(* Logix 5000 AddOnInstructionDefinition export YAI_Assy_166_22_23_EIP_Hz; software revision 17.00 *)

ADD_ON_INSTRUCTION YAI_Assy_166_22_23_EIP_Hz   (* revision 1.0, vendor Yaskawa America, Inc. *)
// YAI Assembly 166 and 22/23
// Help:
// This add-on instruction is for use with input assemblie 166 and output assemblies 116.
// Node_Input_Assy is defined as the node's input assembly integer array.
// Node_Output_Assy is defined as the node's output assembly integer array.
// Torque limit/reference, torque compensation and torque output variables are only available with A1000.
VAR_IN_OUT
   Node_Input_Assy : AB:ETHERNET_MODULE_INT_44Bytes:I:0; {required}   // Input assembly words
   Node_Output_Assy : AB:ETHERNET_MODULE_INT_6Bytes:O:0; {required}   // Output assembly words
END_VAR
VAR_INPUT
   RunFwd : BOOL; {visible}   // Forward run command
   RunRev : BOOL; {visible}   // Reverse run command
   FaultReset : BOOL; {visible}   // Fault reset command
   Freq_Ref : REAL; {visible}   // Frequency reference command in Hz (xx.xx resolution)
   Net_Ref : BOOL;   // Network reference control bit
   Net_Control : BOOL;   // Network start/stop control bit
END_VAR
VAR_OUTPUT
   Running : BOOL; {visible}   // Drive running forward status bit
   ZSP : BOOL; {visible}   // Drive zero speed status bit
   RunningRev : BOOL; {visible}   // Drive running reverse status bit
   Reset : BOOL; {visible}   // Drive reset command status bit
   At_Speed : BOOL; {visible}   // Drive at commanded speed status bit
   Ready : BOOL; {visible}   // Drive ready status bit
   Alarm : BOOL; {visible}   // Drive alarm status bit
   Faulted : BOOL; {visible}   // Drive faulted status bit
   OPE : BOOL;   // OPE alarm/fault present
   UV : BOOL;   // Drive in UV (undervoltage) state status bit
   NetCtrlStatus : BOOL; {visible}   // Drive network run source status bit (1 = source coming from network)
   MFO_1_Status : BOOL; {visible}   // Drive multi-function output 1 (M1-M2 for A/P1000, MA/MB/MC for V1000) status
   MFO_2_Status : BOOL; {visible}   // Drive multi-function output 1 (M3-M4 for A/P1000, P1 for V1000) status
   MFO_3_Status : BOOL; {visible}   // Drive multi-function output 1 (M5-M6 for A/P1000, P2 for V1000) status
   ZSV : BOOL; {visible}   // Drive zero servo completed status bit
   Motor_Speed : REAL; {visible}   // Motor speed in Hz (xx.xx resolution)
   Torque_Actual : REAL; {visible}   // Drive torque output in % (xxx.x resolution)
   PG_Count : INT;   // Encoder feedback count
   Freq_Cmd : REAL; {visible}   // Commanded frequency in Hz (xx.xx resolution)
   Output_Freq : REAL; {visible}   // Drive output frequency in Hz (xx.xx resolution)
   Output_Current : REAL; {visible}   // Drive output current in A (xxx.x resolution)
   Analog_Input_1_Level : REAL;   // Analog input 1 level in % (xxx.x resolution)
   DC_Bus_Volt : INT; {visible}   // DC bus voltage in Vdc (xxx resolution)
   Error_Code : INT;   // Custom input/output error code. Refer to custom error bit to determine which parameter error is pertaining to.
   Custom_In_1 : INT; {visible}   // Custom input 1 - F7-33
   Custom_In_2 : INT; {visible}   // Custom input 2 - F7-34
   Custom_In_3 : INT; {visible}   // Custom input 3 - F7-35
   Custom_In_4 : INT;   // Custom input 4 - F7-36
   Custom_In_5 : INT;   // Custom input 5 - F7-37
   Custom_In_6 : INT;   // Custom input 6 - F7-38
   Custom_In_7 : INT;   // Custom input 7 - F7-39
   Custom_In_8 : INT;   // Custom input 8 -F7-40
   Custom_In_9 : INT;   // Custom input 9 - F7-41
   Custom_In_10 : INT;   // Custom input 10 - F7-42
   Custom_In_1_Error : BOOL;   // Custom input 1 error bit
   Custom_In_2_Error : BOOL;   // Custom input 2 error bit
   Custom_In_3_Error : BOOL;   // Custom input 3 error bit
   Custom_In_4_Error : BOOL;   // Custom input 4 error bit
   Custom_In_5_Error : BOOL;   // Custom input 5 error bit
   Custom_In_6_Error : BOOL;   // Custom input 6 error bit
   Custom_In_7_Error : BOOL;   // Custom input 7 error bit
   Custom_In_8_Error : BOOL;   // Custom input 8 error bit
   Custom_In_9_Error : BOOL;   // Custom input 9 error bit
   Custom_In_10_Error : BOOL;   // Custom input 10 error bit
END_VAR
VAR_INPUT
   Motor_Rated_Torq : REAL;
   Torq_Ref_Limit : REAL;
END_VAR
VAR
   FRef_Convert : DINT;
   FOut_Convert : REAL;
   FOut_Temp : REAL;
   TRef_Convert : INT;
   TComp_Convert : INT;
   TOut_Convert : REAL;
   TOut_Temp : REAL;
   IOut_Temp : REAL;
   IOut_Convert : REAL;
   AO1_Convert : INT;
   AO2_Convert : INT;
   Motor_Speed_Temp : REAL;
   Motor_Speed_Convert : REAL;
   Freq_Cmd_Temp : REAL;
   Freq_Cmd_Convert : REAL;
   AI1_Temp : REAL;
   AI1_Convert : REAL;
   Motor_Torq_Temp : REAL;
END_VAR

ROUTINE Logic   (* ladder *)
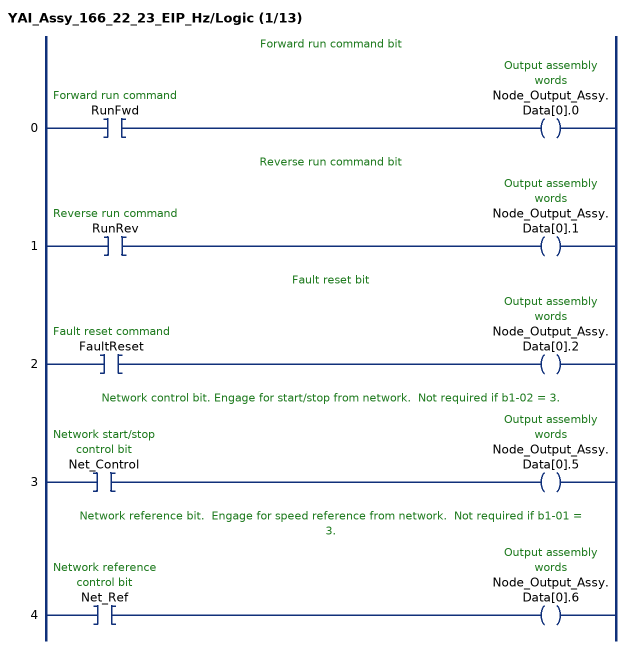
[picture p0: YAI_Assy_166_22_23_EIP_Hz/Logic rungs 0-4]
   // Forward run command bit
   0: XIC(RunFwd)OTE(Node_Output_Assy.Data[0].0);
   // Reverse run command bit
   1: XIC(RunRev)OTE(Node_Output_Assy.Data[0].1);
   // Fault reset bit
   2: XIC(FaultReset)OTE(Node_Output_Assy.Data[0].2);
   // Network control bit. Engage for start/stop from network.  Not required if b1-02 = 3.
   3: XIC(Net_Control)OTE(Node_Output_Assy.Data[0].5);
   // Network reference bit.  Engage for speed reference from network.  Not required if b1-01 = 3.
   4: XIC(Net_Ref)OTE(Node_Output_Assy.Data[0].6);
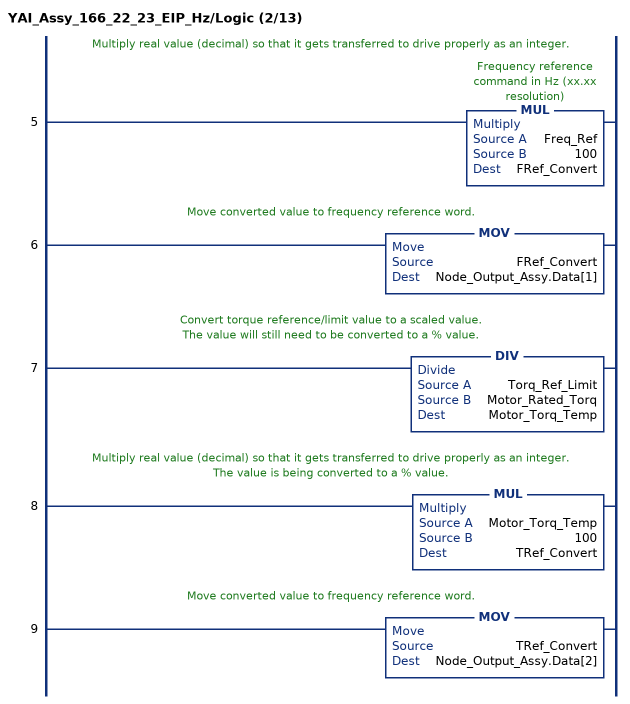
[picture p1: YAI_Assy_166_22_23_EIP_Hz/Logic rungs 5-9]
   // Multiply real value (decimal) so that it gets transferred to drive properly as an integer.
   5: MUL(Freq_Ref,100,FRef_Convert);
   // Move converted value to frequency reference word.
   6: MOV(FRef_Convert,Node_Output_Assy.Data[1]);
   // Convert torque reference/limit value to a scaled value.
   // The value will still need to be converted to a % value.
   7: DIV(Torq_Ref_Limit,Motor_Rated_Torq,Motor_Torq_Temp);
   // Multiply real value (decimal) so that it gets transferred to drive properly as an integer.
   // The value is being converted to a % value.
   8: MUL(Motor_Torq_Temp,100,TRef_Convert);
   // Move converted value to frequency reference word.
   9: MOV(TRef_Convert,Node_Output_Assy.Data[2]);
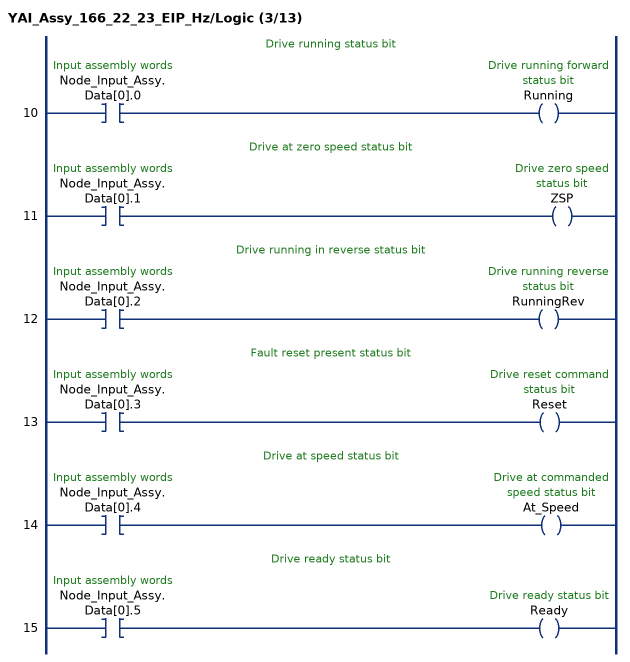
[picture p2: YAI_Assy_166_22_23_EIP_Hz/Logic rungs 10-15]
   // Drive running status bit
   10: XIC(Node_Input_Assy.Data[0].0)OTE(Running);
   // Drive at zero speed status bit
   11: XIC(Node_Input_Assy.Data[0].1)OTE(ZSP);
   // Drive running in reverse status bit
   12: XIC(Node_Input_Assy.Data[0].2)OTE(RunningRev);
   // Fault reset present status bit
   13: XIC(Node_Input_Assy.Data[0].3)OTE(Reset);
   // Drive at speed status bit
   14: XIC(Node_Input_Assy.Data[0].4)OTE(At_Speed);
   // Drive ready status bit
   15: XIC(Node_Input_Assy.Data[0].5)OTE(Ready);
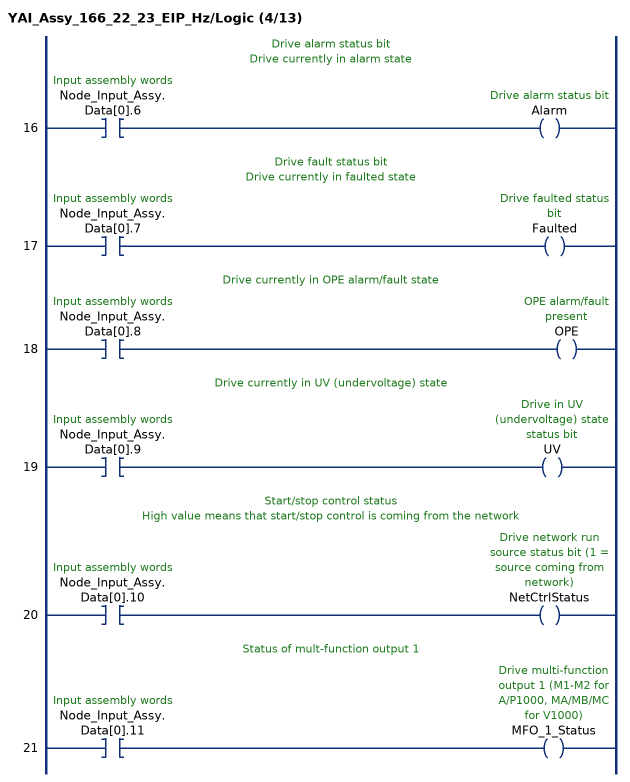
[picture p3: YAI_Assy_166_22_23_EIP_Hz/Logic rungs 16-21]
   // Drive alarm status bit
   // Drive currently in alarm state
   16: XIC(Node_Input_Assy.Data[0].6)OTE(Alarm);
   // Drive fault status bit
   // Drive currently in faulted state
   17: XIC(Node_Input_Assy.Data[0].7)OTE(Faulted);
   // Drive currently in OPE alarm/fault state
   18: XIC(Node_Input_Assy.Data[0].8)OTE(OPE);
   // Drive currently in UV (undervoltage) state
   19: XIC(Node_Input_Assy.Data[0].9)OTE(UV);
   // Start/stop control status
   // High value means that start/stop control is coming from the network
   20: XIC(Node_Input_Assy.Data[0].10)OTE(NetCtrlStatus);
   // Status of mult-function output 1
   21: XIC(Node_Input_Assy.Data[0].11)OTE(MFO_1_Status);
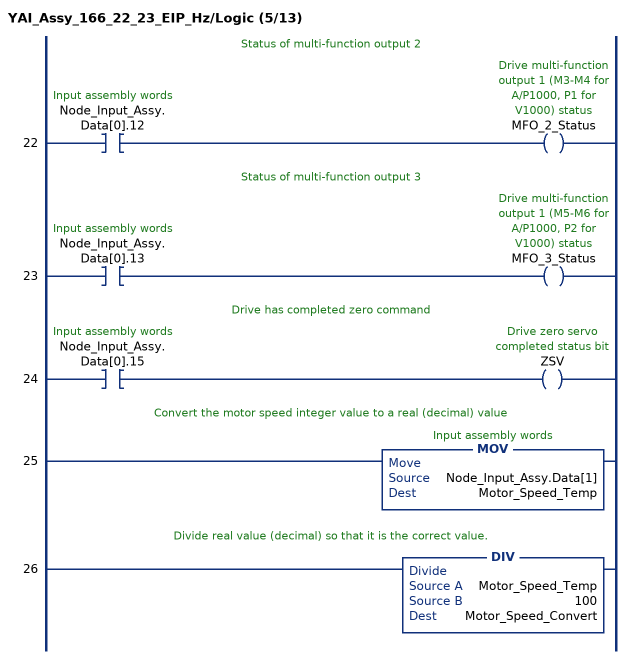
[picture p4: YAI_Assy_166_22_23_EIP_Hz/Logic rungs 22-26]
   // Status of multi-function output 2
   22: XIC(Node_Input_Assy.Data[0].12)OTE(MFO_2_Status);
   // Status of multi-function output 3
   23: XIC(Node_Input_Assy.Data[0].13)OTE(MFO_3_Status);
   // Drive has completed zero command
   24: XIC(Node_Input_Assy.Data[0].15)OTE(ZSV);
   // Convert the motor speed integer value to a real (decimal) value
   25: MOV(Node_Input_Assy.Data[1],Motor_Speed_Temp);
   // Divide real value (decimal) so that it is the correct value.
   26: DIV(Motor_Speed_Temp,100,Motor_Speed_Convert);
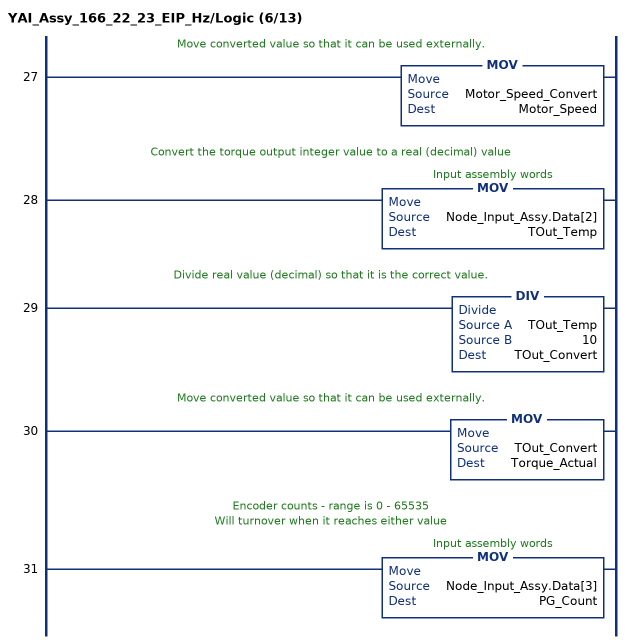
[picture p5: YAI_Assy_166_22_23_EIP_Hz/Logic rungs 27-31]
   // Move converted value so that it can be used externally.
   27: MOV(Motor_Speed_Convert,Motor_Speed);
   // Convert the torque output integer value to a real (decimal) value
   28: MOV(Node_Input_Assy.Data[2],TOut_Temp);
   // Divide real value (decimal) so that it is the correct value.
   29: DIV(TOut_Temp,10,TOut_Convert);
   // Move converted value so that it can be used externally.
   30: MOV(TOut_Convert,Torque_Actual);
   // Encoder counts - range is 0 - 65535
   // Will turnover when it reaches either value
   31: MOV(Node_Input_Assy.Data[3],PG_Count);
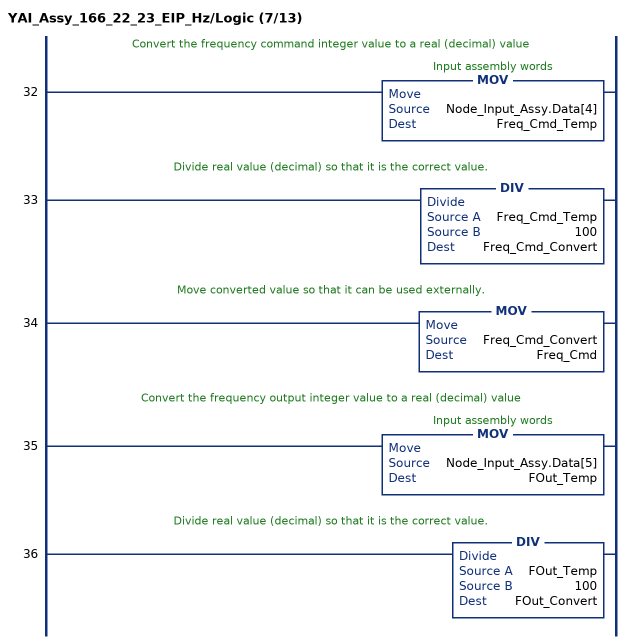
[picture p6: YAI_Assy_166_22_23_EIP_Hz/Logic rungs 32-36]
   // Convert the frequency command integer value to a real (decimal) value
   32: MOV(Node_Input_Assy.Data[4],Freq_Cmd_Temp);
   // Divide real value (decimal) so that it is the correct value.
   33: DIV(Freq_Cmd_Temp,100,Freq_Cmd_Convert);
   // Move converted value so that it can be used externally.
   34: MOV(Freq_Cmd_Convert,Freq_Cmd);
   // Convert the frequency output integer value to a real (decimal) value
   35: MOV(Node_Input_Assy.Data[5],FOut_Temp);
   // Divide real value (decimal) so that it is the correct value.
   36: DIV(FOut_Temp,100,FOut_Convert);
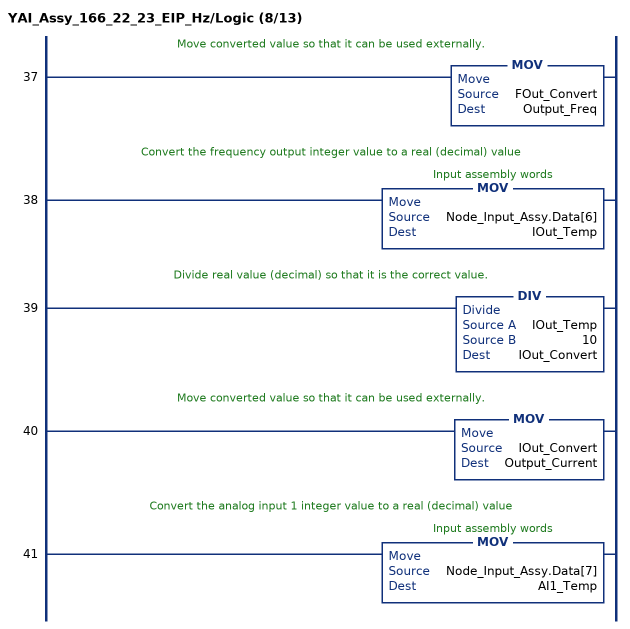
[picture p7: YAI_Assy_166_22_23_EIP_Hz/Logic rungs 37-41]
   // Move converted value so that it can be used externally.
   37: MOV(FOut_Convert,Output_Freq);
   // Convert the frequency output integer value to a real (decimal) value
   38: MOV(Node_Input_Assy.Data[6],IOut_Temp);
   // Divide real value (decimal) so that it is the correct value.
   39: DIV(IOut_Temp,10,IOut_Convert);
   // Move converted value so that it can be used externally.
   40: MOV(IOut_Convert,Output_Current);
   // Convert the analog input 1 integer value to a real (decimal) value
   41: MOV(Node_Input_Assy.Data[7],AI1_Temp);
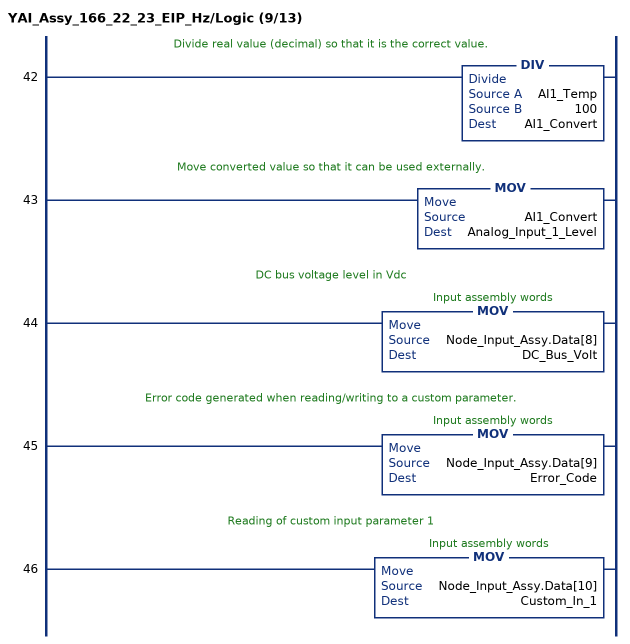
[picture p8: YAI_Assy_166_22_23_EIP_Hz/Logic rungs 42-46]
   // Divide real value (decimal) so that it is the correct value.
   42: DIV(AI1_Temp,100,AI1_Convert);
   // Move converted value so that it can be used externally.
   43: MOV(AI1_Convert,Analog_Input_1_Level);
   // DC bus voltage level in Vdc
   44: MOV(Node_Input_Assy.Data[8],DC_Bus_Volt);
   // Error code generated when reading/writing to a custom parameter.
   45: MOV(Node_Input_Assy.Data[9],Error_Code);
   // Reading of custom input parameter 1
   46: MOV(Node_Input_Assy.Data[10],Custom_In_1);
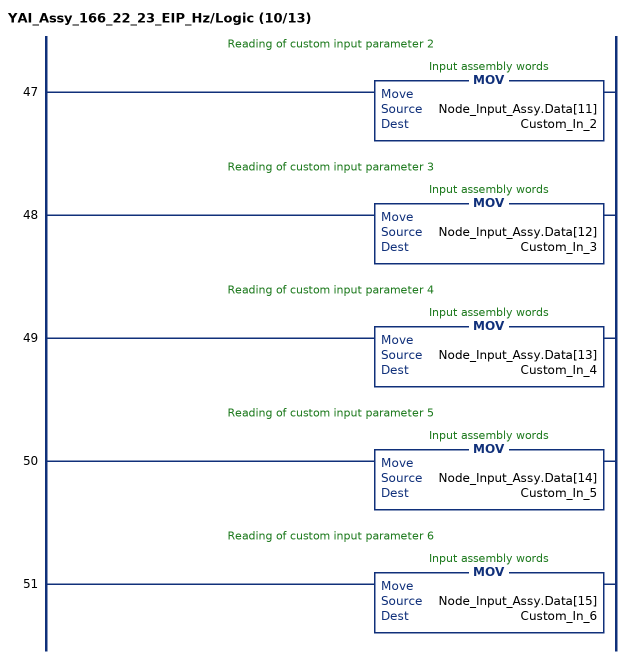
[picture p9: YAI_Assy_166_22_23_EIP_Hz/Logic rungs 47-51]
   // Reading of custom input parameter 2
   47: MOV(Node_Input_Assy.Data[11],Custom_In_2);
   // Reading of custom input parameter 3
   48: MOV(Node_Input_Assy.Data[12],Custom_In_3);
   // Reading of custom input parameter 4
   49: MOV(Node_Input_Assy.Data[13],Custom_In_4);
   // Reading of custom input parameter 5
   50: MOV(Node_Input_Assy.Data[14],Custom_In_5);
   // Reading of custom input parameter 6
   51: MOV(Node_Input_Assy.Data[15],Custom_In_6);
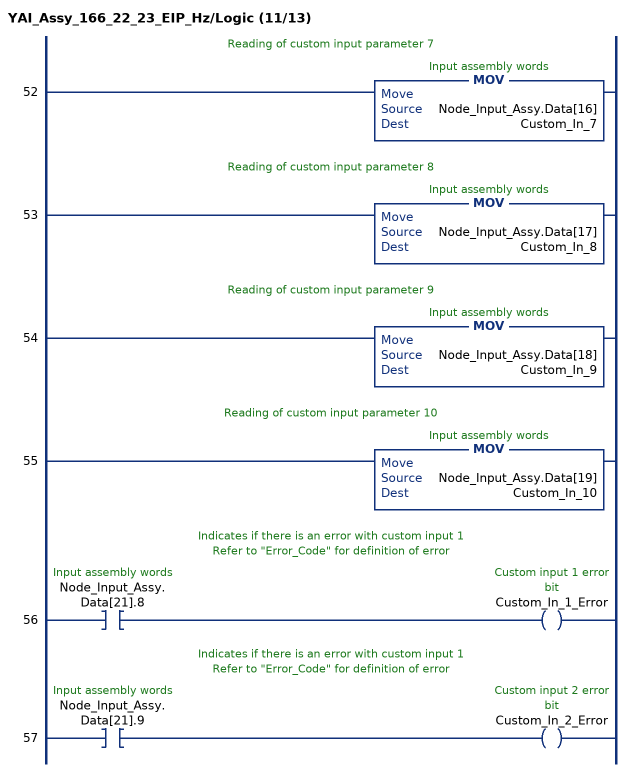
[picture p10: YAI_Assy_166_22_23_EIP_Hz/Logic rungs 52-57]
   // Reading of custom input parameter 7
   52: MOV(Node_Input_Assy.Data[16],Custom_In_7);
   // Reading of custom input parameter 8
   53: MOV(Node_Input_Assy.Data[17],Custom_In_8);
   // Reading of custom input parameter 9
   54: MOV(Node_Input_Assy.Data[18],Custom_In_9);
   // Reading of custom input parameter 10
   55: MOV(Node_Input_Assy.Data[19],Custom_In_10);
   // Indicates if there is an error with custom input 1
   // Refer to "Error_Code" for definition of error
   56: XIC(Node_Input_Assy.Data[21].8)OTE(Custom_In_1_Error);
   // Indicates if there is an error with custom input 1
   // Refer to "Error_Code" for definition of error
   57: XIC(Node_Input_Assy.Data[21].9)OTE(Custom_In_2_Error);
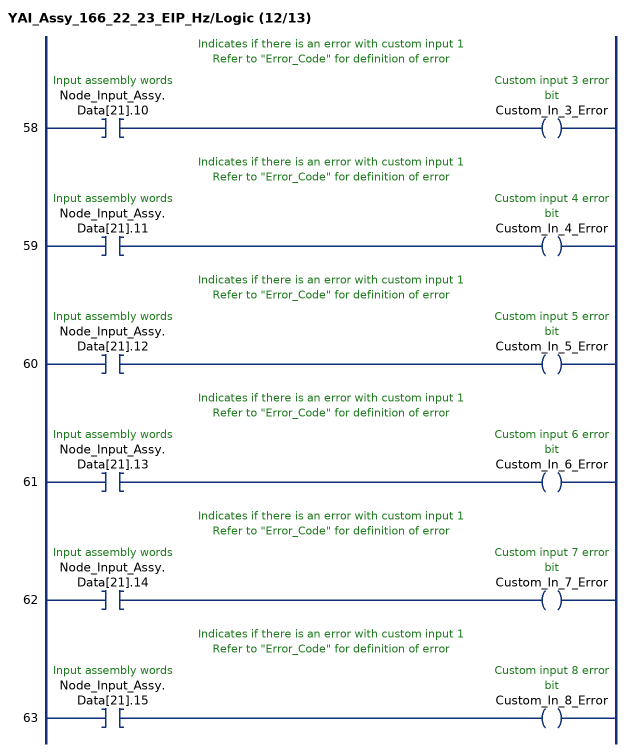
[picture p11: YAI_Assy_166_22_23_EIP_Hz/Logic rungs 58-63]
   // Indicates if there is an error with custom input 1
   // Refer to "Error_Code" for definition of error
   58: XIC(Node_Input_Assy.Data[21].10)OTE(Custom_In_3_Error);
   // Indicates if there is an error with custom input 1
   // Refer to "Error_Code" for definition of error
   59: XIC(Node_Input_Assy.Data[21].11)OTE(Custom_In_4_Error);
   // Indicates if there is an error with custom input 1
   // Refer to "Error_Code" for definition of error
   60: XIC(Node_Input_Assy.Data[21].12)OTE(Custom_In_5_Error);
   // Indicates if there is an error with custom input 1
   // Refer to "Error_Code" for definition of error
   61: XIC(Node_Input_Assy.Data[21].13)OTE(Custom_In_6_Error);
   // Indicates if there is an error with custom input 1
   // Refer to "Error_Code" for definition of error
   62: XIC(Node_Input_Assy.Data[21].14)OTE(Custom_In_7_Error);
   // Indicates if there is an error with custom input 1
   // Refer to "Error_Code" for definition of error
   63: XIC(Node_Input_Assy.Data[21].15)OTE(Custom_In_8_Error);
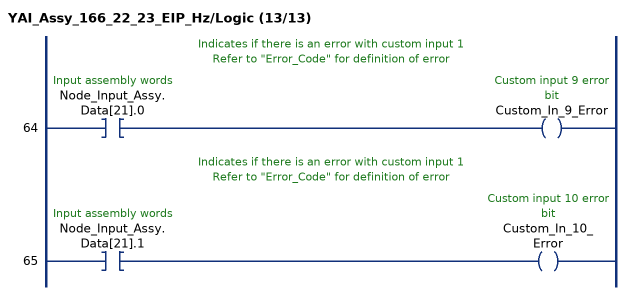
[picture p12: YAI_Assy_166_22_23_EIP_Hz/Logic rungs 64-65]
   // Indicates if there is an error with custom input 1
   // Refer to "Error_Code" for definition of error
   64: XIC(Node_Input_Assy.Data[21].0)OTE(Custom_In_9_Error);
   // Indicates if there is an error with custom input 1
   // Refer to "Error_Code" for definition of error
   65: XIC(Node_Input_Assy.Data[21].1)OTE(Custom_In_10_Error);
END_ROUTINE
END_ADD_ON_INSTRUCTION
